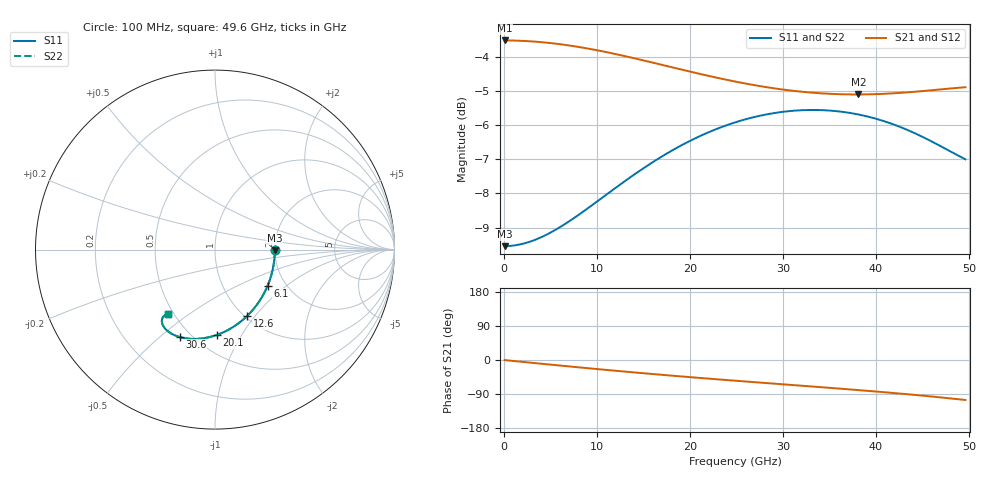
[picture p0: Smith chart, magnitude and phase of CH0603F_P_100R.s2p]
# GHz S RI R 100
! S-Parameters data
! Freq  reS11  imS11  reS21  imS21  reS12  imS12  reS22  imS22
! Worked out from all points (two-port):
!   100 points, 100 MHz to 49.6 GHz, reference 100 ohm
!   highest |S21| = -3.52 dB at 100 MHz (marker M1); lowest = -5.1 dB at 38.1 GHz (marker M2)
!   |S21| within 3 dB of the highest: start of sweep to end of sweep
!   lowest |S11| = -9.5 dB at 100 MHz (marker M3), VSWR 2.00, Z = 200 - j1.55 ohm
!   |S11| at or under -10 dB: nowhere
!   |S22| runs from -9.5 to -5.6 dB; largest |S21 - S12| = 0
!   S11 on the Smith chart (normalised r, x): 100 MHz: 2.00, -0.02; 6.1 GHz: 1.61, -0.75; 12.6 GHz: 1.02, -0.91; 20.1 GHz: 0.64, -0.79; 30.6 GHz: 0.43, -0.58; 49.6 GHz: 0.46, -0.42
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0.1  0.3333 -0.00345  0.6667 -0.00283  0.6667 -0.00283  0.3333 -0.00345
1.6  0.3304 -0.055  0.6645 -0.0452  0.6645 -0.0452  0.3304 -0.055
3.1  0.3225 -0.1058  0.6587 -0.0871  0.6587 -0.0871  0.3225 -0.1058
6.1  0.2926 -0.2023  0.6365 -0.1674  0.6365 -0.1674  0.2926 -0.2023
8.6  0.2552 -0.2748  0.6087 -0.2288  0.6087 -0.2288  0.2552 -0.2748
10.6  0.2187 -0.326  0.5816 -0.2735  0.5816 -0.2735  0.2187 -0.326
12.6  0.1779 -0.3706  0.5512 -0.3139  0.5512 -0.3139  0.1779 -0.3706
14.6  0.1341 -0.4081  0.5182 -0.3498  0.5182 -0.3498  0.1341 -0.4081
16.6  0.0887 -0.4387  0.4837 -0.3813  0.4837 -0.3813  0.0887 -0.4387
20.1  0.00848 -0.4759  0.4214 -0.427  0.4214 -0.427  0.00848 -0.4759
22.6  -0.0468 -0.4908  0.3765 -0.4533  0.3765 -0.4533  -0.0468 -0.4908
25.1  -0.0988 -0.4973  0.332 -0.4751  0.332 -0.4751  -0.0988 -0.4973
27.6  -0.1464 -0.4964  0.2881 -0.4935  0.2881 -0.4935  -0.1464 -0.4964
30.6  -0.1964 -0.4872  0.2358 -0.512  0.2358 -0.512  -0.1964 -0.4872
33.1  -0.2312 -0.4741  0.1921 -0.5251  0.1921 -0.5251  -0.2312 -0.4741
35.6  -0.2592 -0.4572  0.1478 -0.5366  0.1478 -0.5366  -0.2592 -0.4572
38.1  -0.2798 -0.4377  0.102 -0.5464  0.102 -0.5464  -0.2798 -0.4377
41.6  -0.295 -0.4086  0.0336 -0.5567  0.0336 -0.5567  -0.295 -0.4086
43.6  -0.296 -0.3925  -0.00864 -0.56  -0.00864 -0.56  -0.296 -0.3925
45.6  -0.2911 -0.3782  -0.0537 -0.5605  -0.0537 -0.5605  -0.2911 -0.3782
47.6  -0.2802 -0.367  -0.1018 -0.5572  -0.1018 -0.5572  -0.2802 -0.367
49.6  -0.2637 -0.3605  -0.1529 -0.5485  -0.1529 -0.5485  -0.2637 -0.3605
